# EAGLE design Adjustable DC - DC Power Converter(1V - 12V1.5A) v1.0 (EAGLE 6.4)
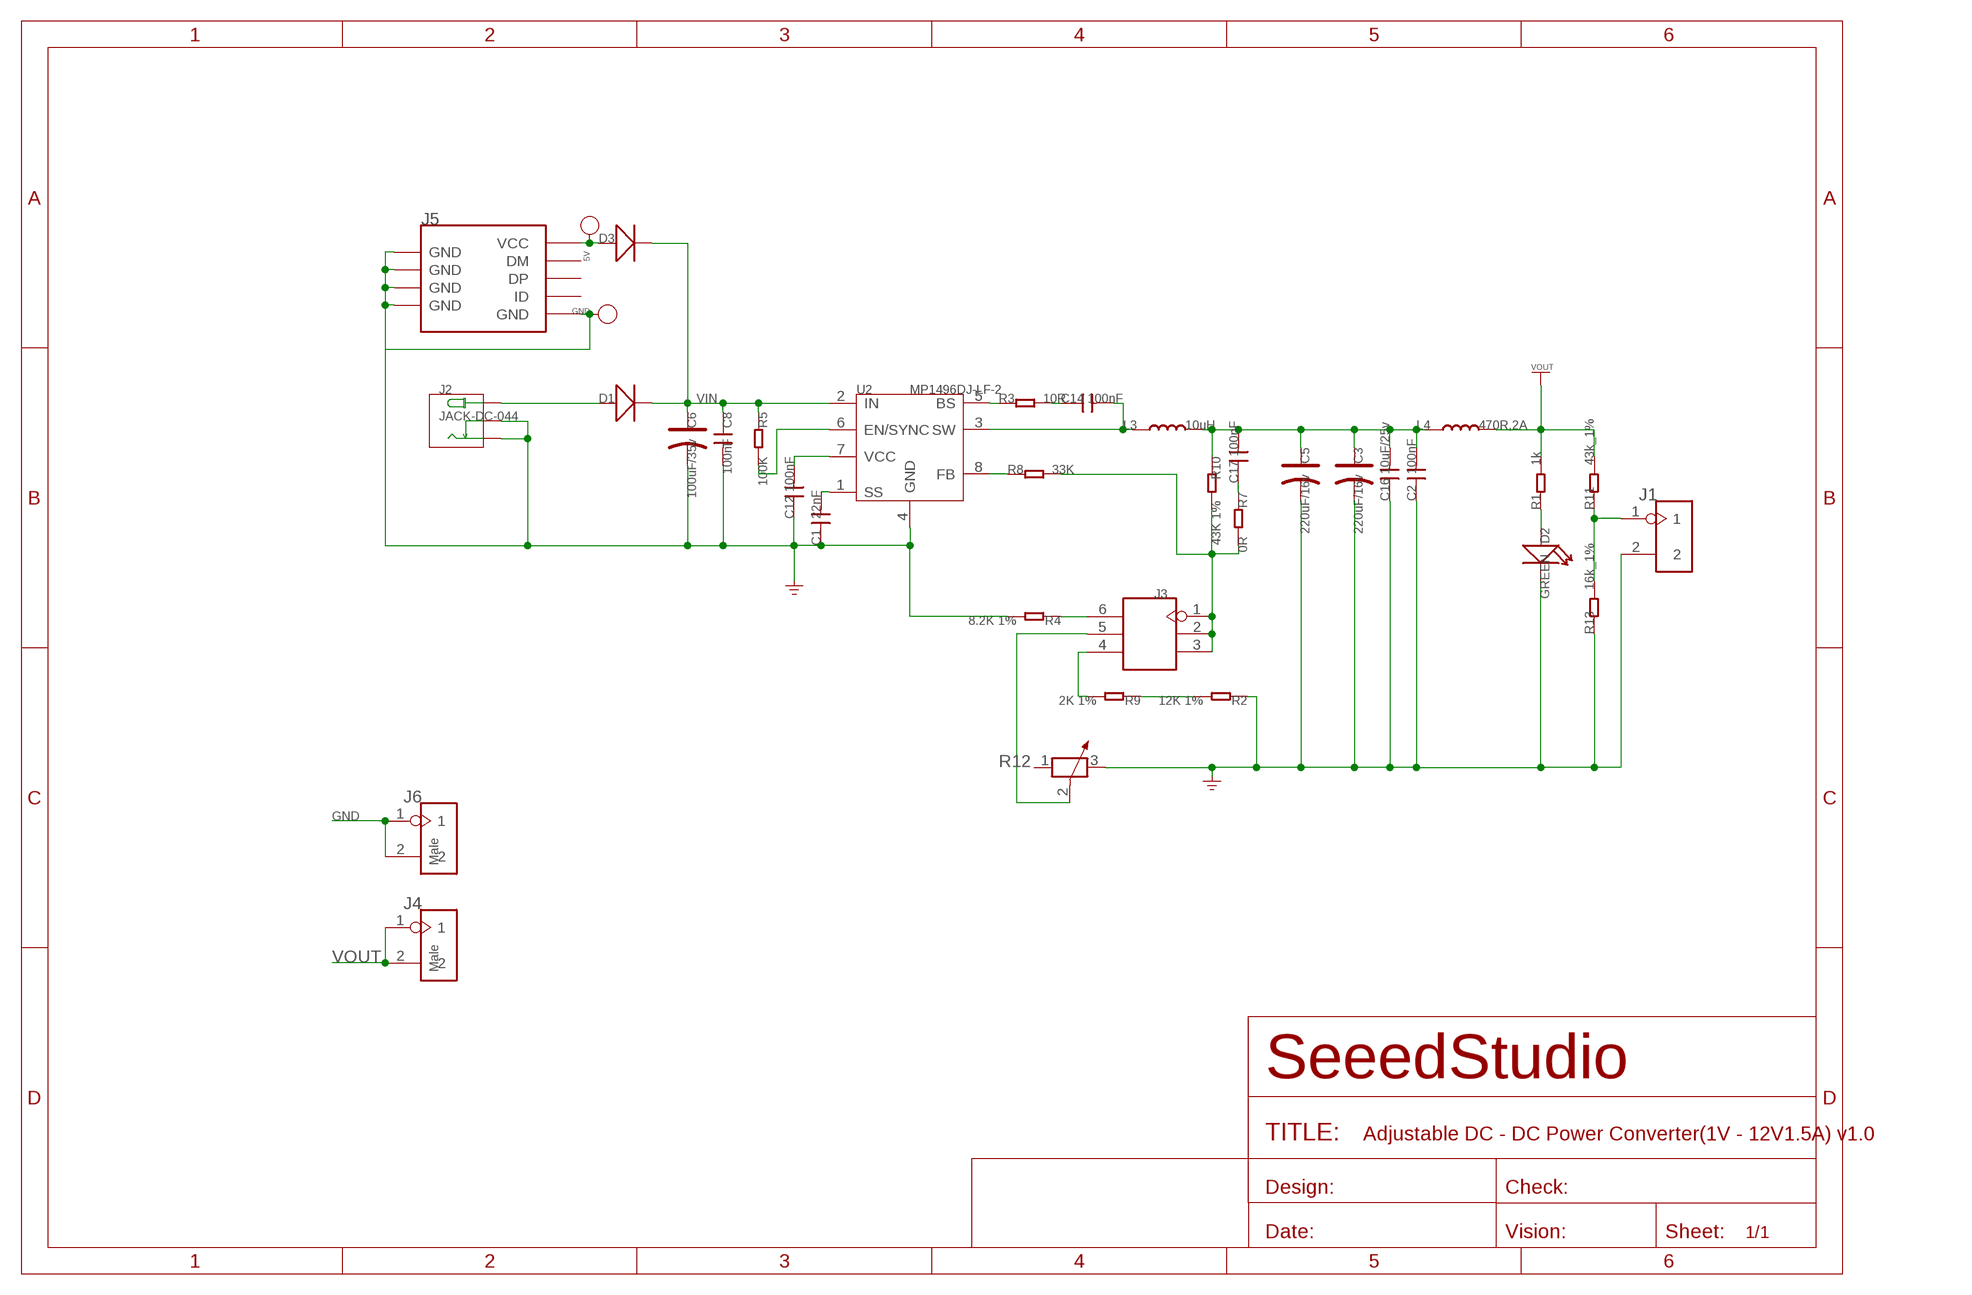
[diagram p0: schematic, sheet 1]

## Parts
5V  PAD-TEST-POINT'4545'  [TP_4545]
C1  22nF  C-0603  [0603]
C2  100nF  C-0603  [0603]
C3  220uF/16v  CAP-ELECTRO-C  [ELECTRO-SMD-C-6MM]
C5  220uF/16v  CAP-ELECTRO-C  [ELECTRO-SMD-C-6MM]
C6  100uF/35v  CAP-ELECTRO-C  [ELECTRO-SMD-C-6MM]
C8  100nF  C-0603  [0603]
C12  100nF  C-0603  [0603]
C14  100nF  C-0603  [0603]
C16  10uF/25v  C-0805  [0805]
C17  100nF  C-0603  [0603]
D1  D'SMA'  [DO-214AC]
D2  GREEN  LED-0603  [D0603]
D3  D'SMA'  [DO-214AC]
GND  PAD-TEST-POINT'4545'  [TP_4545]
J1  HEADER-2P-65/35MIL  [2P-2.54-65/35MIL]
J2  JACK-DC-044  [DC-044]
J3  HEADER-2X3P-65/35MIL  [2X3P-2.54-65/35MIL]
J4  Male  HEADER-2P-65/35MIL  [2P-2.54-65/35MIL]
J5  USB-MINIUSB-5P-MICRO  [MICRO-USB]
J6  Male  HEADER-2P-65/35MIL  [2P-2.54-65/35MIL]
L3  10uH  L'1813'  [1813]
L4  470R,2A  L'0805'  [L0805]
R1  1k  R-0603  [R0603]
R2  12K 1%  R-0603  [R0603]
R3  10R  R-0603  [R0603]
R4  8.2K 1%  R-0603  [R0603]
R5  100K  R-0603  [R0603]
R7  0R  R-0603  [R0603]
R8  33K  R-0603  [R0603]
R9  2K 1%  R-0603  [R0603]
R10  43K 1%  R-0603  [R0603]
R11  43k_1%  R-0603  [R0603]
R12  R-POTENTIOMETER'JML3266W'  [3P-L6.8MM*W4.7MM*H7.3MM]
R13  16k_1%  R-0603  [R0603]
U2  MP1496DJ-LF-2  MP1496DJ  [TSOT23-8]

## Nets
GND: C1.1 C2.1 C3.- C5.- C6.- C8.2 C12.1 C16.1 D2.- GND.T J1.2 J2.- J2.CDN J5.5(GND) J5.S1(GND) J5.S2(GND) J5.S3(GND) J5.S4(GND) J5.S5(GND) J5.S6(GND) J6.1 J6.2 R2.1 R4.2 R12.3 R13.1 U2.4(GND)
N$2: R5.2 U2.6(EN/SYNC)
N$3: C17.1 R7.1
N$4: J3.1 J3.2 J3.3 R7.2 R8.2 R10.2
N$5: J3.4 R9.2
N$6: J3.6 R4.1
N$7: C12.2 U2.7(VCC)
N$8: C1.2 U2.1(SS)
N$9: C2.2 C3.+ C5.+ C16.2 C17.2 L3.2 L4.1 R10.1
N$10: R3.1 U2.5(BS)
N$11: C14.1 R3.2
N$12: C14.2 L3.1 U2.3(SW)
N$13: R2.2 R9.1
N$14: R8.1 U2.8(FB)
N$15: J3.5 R12.2
N$16: J1.1 R11.1 R13.2
N$19: D2.+ R1.1
N$21: 5V.T D3.1(+) J5.1(VCC)
N$22: D1.1(+) J2.+
VIN: C6.+ C8.1 D1.2(-) D3.2(-) R5.1 U2.2(IN)
VOUT: J4.1 J4.2 L4.2 R1.2 R11.2
Unconnected: J5.2(DM) J5.3(DP) J5.4(ID) R12.1

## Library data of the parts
5V GND = Discrete:PAD-TEST-POINT; PARTNO: DNP
C1 C2 C8 C12 C14 C16 C17 = Discrete:C*: Ceramic Capacitors
C3 C5 C6 = Discrete:CAP*: Electrolytic Capacitors,Tantalum Capacitors and Super Capacitors
D1 D3 = Discrete:D*
D2 = Discrete:LED*
J1 J4 J6 = Connector:HEADER-2P
J2 = Connector :JACK-DC-044
J3 = Connector:HEADER-2X3P
J5 = Connector:USB-MINIUSB-5P
L3 L4 = Discrete:L*
R1-R5 R7-R11 R13 = Discrete:R*
R12 = Discrete:R-POTENTIOMETER*: Potentiometer
U2 = template:MP1496DJ: High-Efficiency,2A，16V,500kHz Synchronous,Step-Down Converter http://html.alldatasheetcn.com/html-pdf/551584/MPS/MP1496DJ/55/1/MP1496DJ.html

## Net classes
0 default: width 0.003 mm, drill 0.254 mm, clearance 0.152 mm

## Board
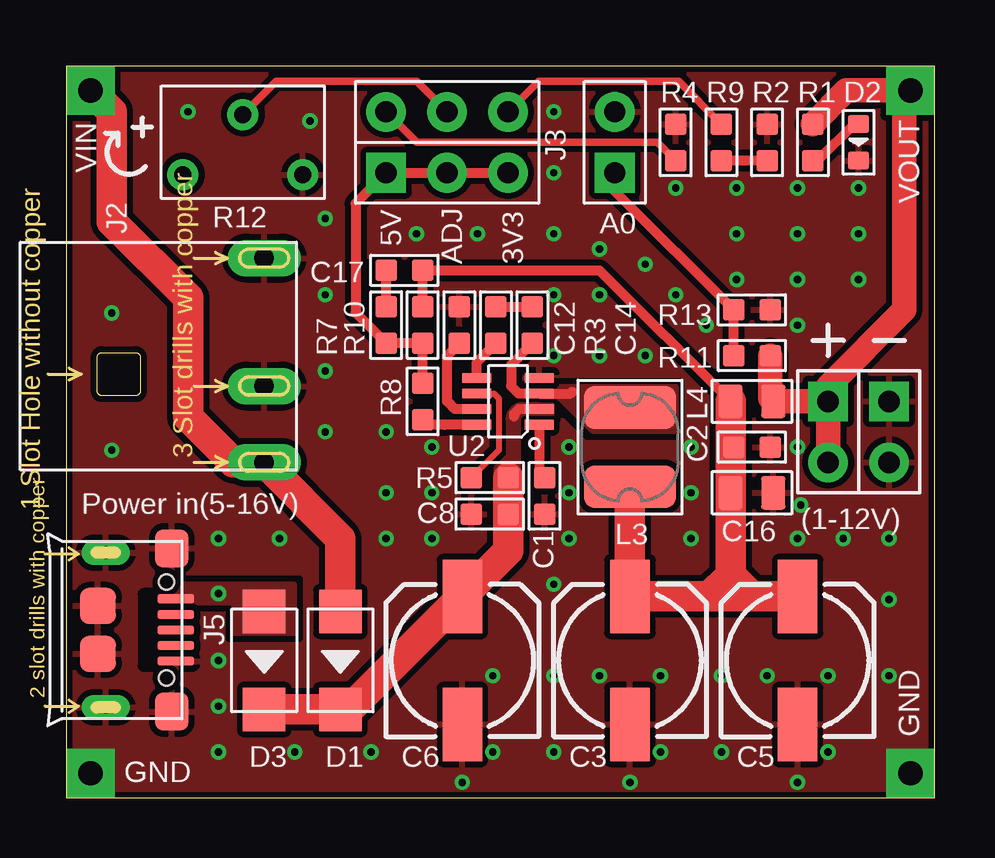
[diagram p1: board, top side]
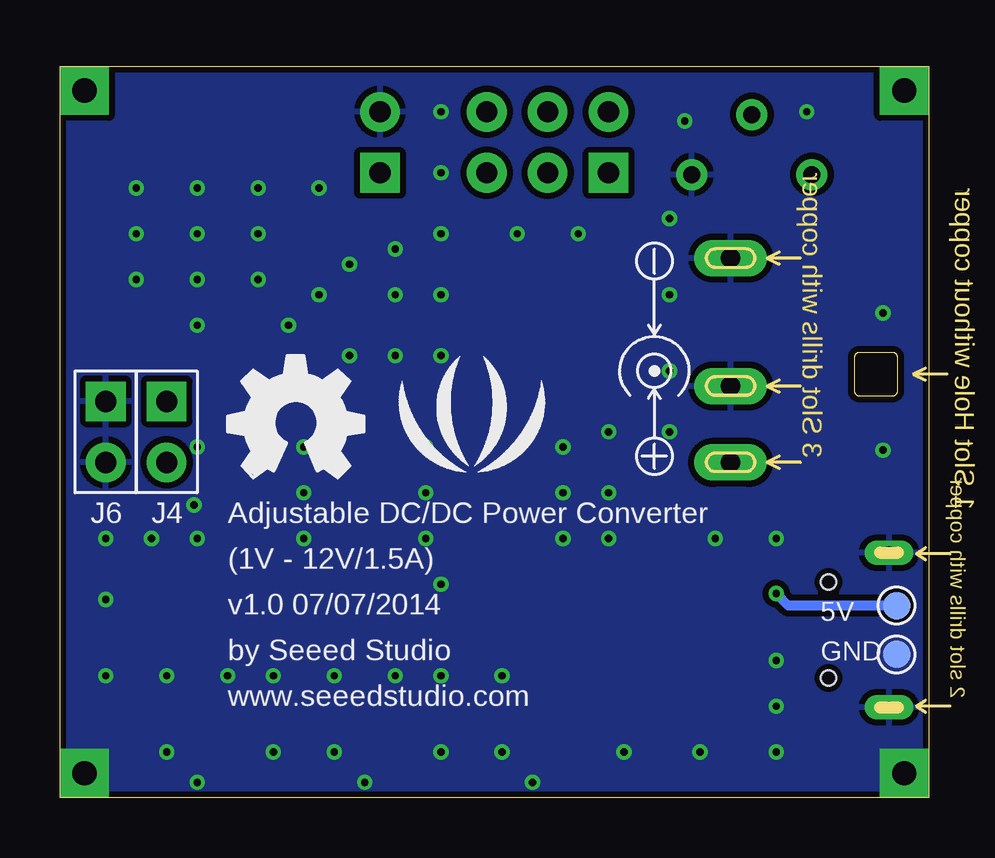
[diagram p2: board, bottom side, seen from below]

Size 36.2 x 30.48 mm. Coordinates in mm from the lower left corner, seen from the top.
Outline: 0,0 36.2,0 36.2,30.48 0,30.48 0,0
Copper layers (1*16): Top 0.035mm / dielectric 1.5mm / Bottom 0.035mm
Design rules "SeeedStudio_rule_no_angle_090911 *": minimum track width 6mil, minimum drill 12mil, track to track 6mil, track to pad 6mil, pad to pad 6mil, via to via 6mil, smd to smd 0mil, copper to edge 10mil, drill to drill 10mil, minimum pad ring 10mil, minimum via ring 6mil, stop-mask expansion 2mil, vias tented up to drill 25mil, thermal gap 10mil

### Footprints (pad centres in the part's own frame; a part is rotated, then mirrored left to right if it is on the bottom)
TP_4545 = smd 1.143 x 1.143: T 0,0
0603 = smd 0.889 x 0.889: 1 -0.762,0; 2 0.762,0
ELECTRO-SMD-C-6MM = smd 3.048 x 1.651: + 2.667,0; - -2.667,0
0805 = smd 1.016 x 1.397: 1 -0.889,0; 2 0.889,0
DO-214AC = smd 1.8 x 1.77: 1 -2.042,0; 2 2.042,0
D0603 = smd 0.762 x 0.889: + -0.762,0; - 0.762,0
2P-2.54-65/35MIL = drill 0.889 pad 1.651 square: 1 0,1.27 | drill 0.889 pad 1.651: 2 0,-1.27
DC-044 = drill 0.813 pad 1.524 long: + 3.175,10.16; - -5.334,10.16; CDN 0,10.16
2X3P-2.54-65/35MIL = drill 0.889 pad 1.651 square: 1 -1.27,2.54 | drill 0.889 pad 1.651: 2 -1.27,0; 3 -1.27,-2.54; 4 1.27,-2.54; 5 1.27,0; 6 1.27,2.54
MICRO-USB = smd 0.381 x 1.524: 1 -1.3,-0.25; 2 -0.65,-0.25; 3 0,-0.25; 4 0.65,-0.25; 5 1.3,-0.25 | smd 1.6 x 1.397: S1 -3.4,-0.427; S6 3.4,-0.427 | drill 0.508 pad 1.016 long: S2 -3.226,-3.175; S5 3.226,-3.175 | smd 1.5 x 1.5: S3 -1,-3.5; S4 1,-3.5 | hole 0.635: -2,-0.65; 2,-0.65
1813 = smd 1.778 x 3.81: 1 -1.651,0; 2 1.651,0
L0805 = smd 1.016 x 1.397: 1 -0.889,0; 2 0.889,0
R0603 = smd 0.889 x 0.889: 1 -0.762,0; 2 0.762,0
3P-L6.8MM*W4.7MM*H7.3MM = drill 0.7 pad 1.3: 1 -2.5,-1.35; 2 0,1.15; 3 2.5,-1.35
TSOT23-8 = smd 0.4 x 1.2: 1 -0.975,-1.3; 2 -0.325,-1.3; 3 0.325,-1.3; 4 0.975,-1.3; 5 0.975,1.3; 6 0.325,1.3; 7 -0.325,1.3; 8 -0.975,1.3

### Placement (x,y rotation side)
5V  1.33,8 0 bottom
C1  19.94,12.57 90 top
C2  28.57,14.61 180 top
C3  23.5,5.71 90 top
C5  30.48,5.71 90 top
C6  16.51,5.71 90 top
C8  17.65,11.81 180 top
C12  16.38,19.68 270 top
C14  19.43,19.68 270 top
C16  28.57,12.7 180 top
C17  14.1,21.97 0 top
D1  11.43,5.71 270 top
D2  33.02,27.3 270 top
D3  8.26,5.71 270 top
GND  1.33,5.97 0 bottom
J1  22.86,27.3 180 top
J2  -1.91,17.14 270 top
J3  15.88,27.3 90 top
J4  31.75,15.24 0 bottom
J5  4.83,6.99 270 top
J6  34.29,15.24 0 bottom
L3  23.5,14.61 270 top
L4  28.57,16.51 0 top
R1  31.11,27.3 90 top
R2  29.21,27.3 270 top
R3  17.91,19.68 90 top
R4  25.4,27.3 90 top
R5  17.65,13.34 180 top
R7  13.34,19.68 270 top
R8  14.86,16.51 90 top
R9  27.3,27.3 90 top
R10  14.86,19.68 270 top
R11  28.57,18.41 0 top
R12  7.37,27.3 0 top
R13  28.57,20.32 180 top
U2  18.41,16.51 90 top
U$4  [OSHW_FILLX200_NOTEXT]  29.21,13.34 0 bottom
U$5  [LOGO_SILK]  19.05,15.24 0 bottom

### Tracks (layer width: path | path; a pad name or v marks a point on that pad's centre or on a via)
GND  (via drill 0.3 pad 0.64, 1.02 pad 2.03)
  other vias: 1.02,1.02 35.18,1.02 20.32,18.41 22.23,18.41 24.13,18.41 15.24,10.79 15.24,12.7 15.24,14.61 6.35,5.71 6.35,3.81 6.35,1.91 20.95,10.79 20.95,14.61 20.95,12.7 26.04,14.61 26.04,10.79 30.48,14.61 30.61,12.19 32.38,10.79 30.48,10.79 31.75,1.91 30.48,0.64 27.3,1.91 23.5,0.64 20.32,1.91 17.78,1.91 16.51,0.64 12.7,1.91 9.53,1.91 24.77,1.91 22.23,20.95 20.32,20.95 26.67,19.68 25.4,20.95 24.13,22.23 25.4,25.4 33.02,25.4 30.48,25.4 27.94,25.4 27.94,21.59 30.48,21.59 30.48,23.5 27.94,23.5 20.32,23.5 20.32,26.04 22.23,22.86 31.75,5.08 29.21,5.08 24.77,5.08 22.23,5.08 17.78,5.08 20.32,8.89 27.3,5.08 20.32,5.08 33.02,23.5 33.02,21.59 10.16,28.19 10.79,24.13 10.79,20.95 10.79,17.78 10.79,15.24 13.34,15.24 13.34,12.7 13.34,10.79 8.89,10.79 6.35,10.79 34.29,10.79 34.29,8.26 17.14,23.5 14.61,23.5 20.32,28.57 34.29,5.08 26.04,12.7 5.08,28.57 1.91,20.19 1.91,14.48 30.48,19.68
  pour Top (isolate 0.254, rank 6): 0,30.48 36.2,30.48 36.2,0 0,0
  pour Bottom (isolate 0.254, rank 6): 0,30.48 36.2,30.48 36.2,0 0,0
N$2
  Top 0.254: U2.6 17.84,16.84 18.03,16.64 18.03,14.48 R5.2
N$3
  Top 0.406: R7.1 C17.1
N$4
  Top 0.406: J3.3 J3.2 J3.1 12.06,24.77 12.06,20.19 R7.2 R10.2 R8.2
N$5
  Top 0.305: J3.4 19.68,29.84 25.53,29.84 R9.2
N$6
  Top 0.305: R4.1 24.64,27.3 14.61,27.3 J3.6
N$7
  Top 0.406: U2.7 16.2,16.18 15.88,16.51 15.88,18.41 C12.2
N$8
  Top 0.406: 20.07,13.34 C1.2 19.71,13.56 U2.1
N$9
  Top 0.406: R10.1 C17.2 22.23,21.97 L4.1
  Top 0.61: C2.2 27.81,14.48 27.69,14.35
  Top 1.016: 27.69,8.51 27.56,8.38
  Top 1.27: L3.2 C3.+ 26.8,8.38 | C5.+ 28.57,8.38 | 28.57,8.38 27.56,8.38 26.8,8.38 | 27.69,9.27 C16.2 27.69,14.35 L4.1 | 27.69,9.27 27.69,8.51 | 26.8,8.38 27.69,9.27 | 27.69,9.27 28.57,8.38
N$10
  Top 0.406: U2.5 17.11,18.13 R3.1
N$11
  Top 0.406: R3.2 C14.1
N$12
  Top 0.406: 22.92,16.84 L3.1 | C14.2 18.54,18.03 18.54,17.14 18.85,16.84 19.34,16.84 U2.3 21.03,16.84 21.08,16.89
  pour Top (isolate 0.254, no thermals): 19.05,17.14 25.4,17.14 25.4,15.24 21.97,15.24 20.57,16.64 19.05,16.64
N$13
  Top 0.406: R2.2 R9.1
N$14
  Top 0.203: 15.45,15.54 15.07,15.54 R8.1
  Top 0.406: U2.8 15.77,15.54 15.45,15.54 14.95,15.54 14.86,15.62
N$15
  Top 0.305: J3.5 14.61,29.84 8.76,29.84 R12.2
N$16
  Top 0.406: R11.1 R13.2 22.86,25.27 J1.1
N$19
  Top 0.406: R1.1 31.3,26.54 32.83,28.07 D2.+
N$21  (via drill 0.3 pad 0.64)
  Top 0.406: v6.35,8.51 6.48,8.51
  Bottom 0.406: 5V.T 5.84,8 v6.35,8.51
  pour Top (isolate 0.254, no thermals): 3.81,8.13 6.99,8.13 6.99,6.86 9.53,6.86 9.53,8.89 3.81,8.89
N$22  (via drill 1.02 pad 2.03)
  Top 1.27: D1.1 11.43,10.79 J2.+ 6.97,13.97 5.08,15.86 5.08,20.83 1.91,24 1.91,28.57 v1.02,29.46
VIN
  Top 0.406: U2.2 18.85,16.18 18.67,16 18.67,15.88
  Top 1.27: D3.2 D1.2 11.8,3.67 C6.+ 18.41,10.29 C8.1 R5.1
  pour Top (isolate 0.152, rank 2, no thermals): 20.26,15.88 20.26,16.38 19.06,16.38 arc45 18.61,16.2 18.6,16.19 arc45 18.41,15.74 18.41,14.22 17.91,13.72 17.91,13.34 18.86,13.34 18.86,15.88
VOUT  (via drill 1.02 pad 2.03)
  Top 1.016: J4.1 L4.2 29.34,16.64 R11.2 | J4.2 J4.1 | R1.2 32.51,29.46 34.8,29.46 | v35.18,29.46 34.8,29.46 | 34.8,29.46 34.92,29.34 34.92,20.32 31.75,17.14 J4.1

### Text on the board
tPlace: VIN | VOUT | 5V | A0 | ADJ | 3V3 | Power in(5-16V) | (1-12V) | GND | GND
bPlace: Adjustable DC/DC Power Converter | (1V - 12V/1.5A) | v1.0 07/07/2014 | by Seeed Studio | www.seeedstudio.com
Reference: J8 | JST | MINIUSB | 1K | 1K | J1 | GREEN | GREEN | J6 | J2 | 10U | 10N | J7 | J3 | 10U | 100N | J5 | J4 | 100U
